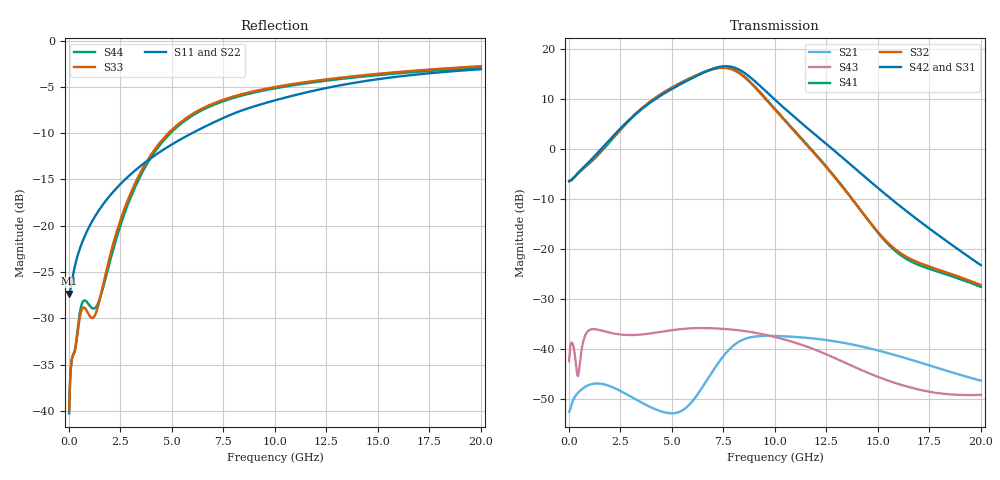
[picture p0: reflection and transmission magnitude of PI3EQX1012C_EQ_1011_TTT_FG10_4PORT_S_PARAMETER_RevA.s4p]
! NPort=4 DATA=2000 NOISE=0 GROUPDELAY=0 COMPLEX_DATAFORMAT=POLAR
! NumOfBlock=1 NumOfParam=0
! .MODEL Smodel S TSTONEFILE=PI3EQX1012C_EQ_1011_TTT_FG10_4PORT_S_PARAMETER_RevA.s4p TYPE=S
!  -- The above .MODEL line can be used for the S element in the netlist.
! The s parameter is extracted from the linear redriver, it is not bi-directional; only s(4,1)s(4,2) and s(3,1)s(3,2)
! should be the insertion loss
!Port definition:
!Port1 = input+
!Port2 = input-
!Port3 = output+
!Port4 = output-
# Hz S MA R  50
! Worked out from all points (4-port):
!   2000 points, 10 MHz to 20 GHz, reference 50 ohm
!   strongest paths, dB at 10 MHz, 5.01 GHz, 10.01 GHz, 15.01 GHz, 20 GHz:
!     S42: -6.4, 12.0, 9.8, -7.8, -23.2
!     S31: -6.4, 12.0, 9.7, -8.0, -23.6
!     S32: -6.4, 12.3, 7.8, -16.6, -27.2
!     S41: -6.4, 12.3, 8.0, -16.8, -27.5
!     S43: -42.4, -36.2, -37.5, -45.5, -49.1
!     S21: -52.4, -52.8, -37.3, -40.2, -46.3
!   lowest |S11| = -27.3 dB at 10 MHz (marker M1), VSWR 1.09, Z = 45.9 - j0.123 ohm
!   |S11| at or under -10 dB: start of sweep to 5.98 GHz
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1e7  0.04301 -178.2  0.002379 1.5  0.0008102 -0.5  0.0008039 -0.5
     0.002388 1.5  0.04109 -178.1  0.000927 -0.5  0.0009197 -0.5
     0.4786 0.2  0.4777 -179.7  0.01016 -4.0  0.007598 -25.7
     0.4772 -179.7  0.4795 0.2  0.007614 -25.8  0.009722 -4.0
4.06e9  0.2352 -124.3  0.002607 1.2  0.0003851 -56.6  0.0003833 -57.0
        0.002591 1.2  0.2388 -123.2  0.0004378 -57.3  0.0004357 -57.6
        3.014 -61.8  3.091 127.1  0.2488 -83.2  0.01354 34.3
        3.073 127.8  3.012 -60.2  0.0145 31.2  0.2409 -82.9
5.74e9  0.3062 -123.7  0.002774 50.9  0.0002783 -58.3  0.0002771 -59.2
        0.002668 48.8  0.3112 -123.0  0.0003156 -59.3  0.0003143 -60.2
        4.777 -130.6  4.909 58.0  0.3847 -99.4  0.01642 9.6
        4.926 58.3  4.798 -128.7  0.0161 7.0  0.3769 -99.2
7.03e9  0.3615 -124.2  0.006597 65.7  0.0002403 -55.9  0.0002382 -57.2
        0.006262 66.5  0.3668 -123.7  0.0002711 -57.1  0.0002689 -58.4
        6.325 165.5  6.278 -6.6  0.458 -109.4  0.01675 -10.6
        6.329 -6.7  6.362 167.6  0.01619 -11.3  0.4497 -109.3
8.08e9  0.4068 -125.7  0.01162 44.2  0.0002253 -54.3  0.0002223 -55.8
        0.01126 45.8  0.4127 -125.2  0.0002525 -55.6  0.0002492 -57.1
        6.401 101.0  6.013 -71.6  0.502 -115.7  0.01594 -25.0
        6.083 -72.0  6.44 103.3  0.01561 -25.1  0.4934 -115.6
9.27e9  0.4507 -127.9  0.01376 14.3  0.000216 -53.8  0.0002121 -55.4
        0.01354 15.8  0.4575 -127.4  0.0002405 -55.0  0.0002363 -56.5
        4.252 34.0  3.648 -138.3  0.5408 -121.3  0.01456 -39.3
        3.703 -139.2  4.279 36.5  0.01433 -39.8  0.5321 -121.2
2e10  0.7005 -144.6  0.00491 -75.1  0.0001464 -72.3  0.0001413 -73.8
      0.00486 -74.0  0.7155 -144.4  0.0001623 -72.1  0.0001566 -73.8
      0.0657 102.4  0.04375 29.1  0.7272 -143.5  0.003591 -51.5
      0.04193 27.4  0.06906 107.1  0.00351 -48.8  0.7152 -143.3
